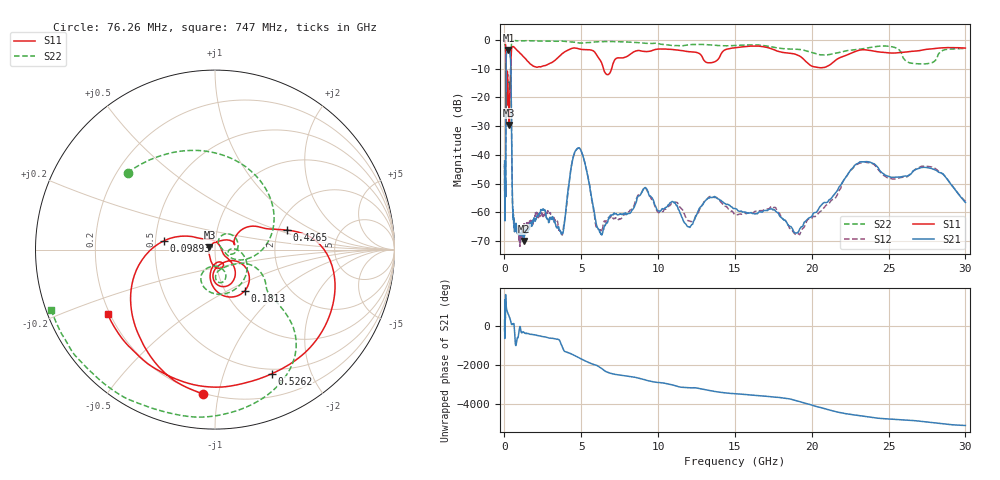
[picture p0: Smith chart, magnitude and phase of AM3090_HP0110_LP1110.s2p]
! Date/Time: Thu, Feb 28, 2019 2:00 PM
! Network Analyzer: Agilent Technologies E8364B Rev: A.07.50.67
! Sweep from 0.010 to 30.000 GHz, 1601 Points, Sweep Type: LOG
! Power Supply: 5.023 V, 0.002 A
# Hz S DB R 50
!freq MagS11 AngS11 MagS21 AngS21 MagS12 AngS12 MagS22 AngS22
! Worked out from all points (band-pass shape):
!   1601 points, 10 MHz to 30 GHz, reference 50 ohm
!   highest |S21| = -3.49 dB at 259.9 MHz (marker M1); lowest = -69.9 dB at 1.257 GHz (marker M2)
!   |S21| within 3 dB of the highest: 113.2 MHz to 397 MHz (283.8 MHz wide, 111 % of centre)
!   lowest |S11| = -29.6 dB at 312.7 MHz (marker M3), VSWR 1.07, Z = 47 + j1.14 ohm
!   |S11| at or under -10 dB: 98.39 MHz to 410.1 MHz (311.7 MHz wide, 123 % of centre); 6.447 GHz to 6.976 GHz (528.7 MHz wide, 7.88 % of centre)
!   |S22| runs from -29.4 to -0.2 dB; largest |S21 - S12| = 0.014
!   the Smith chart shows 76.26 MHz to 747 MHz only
!   S11 on the Smith chart (normalised r, x): 76.26 MHz: 0.20, -0.90; 98.93 MHz: 0.56, +0.06; 181.3 MHz: 1.23, -0.61; 426.5 MHz: 2.22, +0.58; 526.2 MHz: 0.45, -1.46; 747 MHz: 0.19, -0.27
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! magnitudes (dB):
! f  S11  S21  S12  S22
! 10 MHz  -0.3  -42.1  -43.5  -0.7
! 38.04 MHz  -0.5  -62.7  -60.6  -1.6
! 76.26 MHz  -1.9  -53.6  -52.7  -3.8
! 98.93 MHz  -10.8  -17.6  -17.6  -11.6
! 107.2 MHz  -29.4  -8.6  -8.5  -28.6
! 144.7 MHz  -21.3  -4.0  -4.0  -22.3
! 181.3 MHz  -11.0  -3.7  -3.6  -12.9
! 259.9 MHz  -21.1  -3.5  -3.4  -19.1
! 312.7 MHz  -29.6  -3.8  -3.8  -15.9
! 426.5 MHz  -7.7  -12.9  -12.9  -5.8
! 526.2 MHz  -2.4  -56.7  -57.2  -0.5
! 550.5 MHz  -2.4  -59.0  -59.5  -0.4
! 747 MHz  -3.1  -65.1  -65.5  -0.3
! 1.257 GHz  -6.0  -69.9  -64.1  -0.3
! 2.084 GHz  -9.5  -61.9  -60.0  -0.3
! 3.723 GHz  -5.0  -67.6  -67.0  -0.4
! 4.805 GHz  -3.1  -37.6  -37.6  -1.0
! 6.171 GHz  -6.6  -66.2  -66.1  -0.6
! 7.926 GHz  -5.9  -60.8  -60.5  -0.7
! 19.12 GHz  -5.4  -66.9  -67.4  -3.3
! 23.48 GHz  -3.4  -42.4  -42.5  -2.9
! 30 GHz  -2.8  -56.5  -56.2  -3.0
